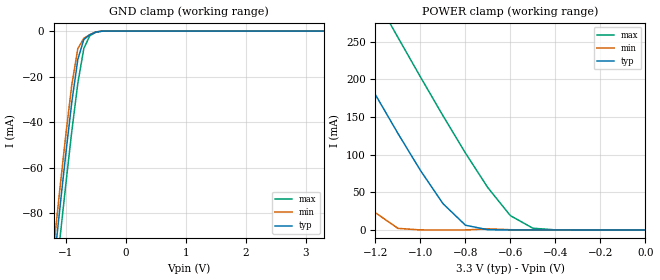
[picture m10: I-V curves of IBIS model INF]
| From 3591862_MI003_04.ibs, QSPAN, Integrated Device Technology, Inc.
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|   Model INF
[Model]   INF
Model_type   Input
Polarity   Non-Inverting
Vinl =   0.8000V
Vinh =   2.0000V
C_comp   5.0000pF   5.0000pF   5.0000pF
[Temperature Range]   27.0000   0.000   70.0000
[Voltage Range]   3.3000V   3.0000V   3.5000V
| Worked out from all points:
|   GND clamp passes 1 mA (typ) near -0.55 V on its own axis
|   POWER clamp passes 1 mA (typ) near -0.71 V on its own axis
[GND_clamp]
| voltage   I(typ)   I(min)   I(max)
-3.3V     -657.8mA   -650mA     -670.4mA
-1.2V     -102.9mA   -94.41mA   -116.5mA
-1.1V     -77.92mA   -69.49mA   -91.49mA
-1V       -53.74mA   -45.47mA   -67.11mA
-900mV    -31.1mA    -23.5mA    -43.83mA
-800mV    -12.43mA   -7.699mA   -22.86mA
-700mV    -3.677mA   -3.173mA   -7.646mA
-600mV    -1.604mA   -1.565mA   -2.006mA
-500mV    -425uA     -358.5uA   -542.4uA
-300mV    -1.113uA   -303.8nA   -5.045uA
3.3V      99.47pA    10.09nA    -13.74uA
[POWER_clamp]
| voltage   I(typ)   I(min)   I(max)
-3.3V     1.331A     1.151A     1.463A
-1.7V     447.3mA    270.6mA    579.2mA
-1.4V     285.1mA    113.5mA    416mA
-1.3V     231.9mA    64.74mA    362.1mA
-1.2V     179.4mA    22.86mA    308.5mA
-1.1V     128mA      2.107mA    255.4mA
-900mV    34.94mA    634.8nA    151.6mA
-800mV    6.306mA    9.188nA    102mA
-700mV    263.5uA    1.485mA    55.91mA
-600mV    6.458uA    324.3uA    18.95mA
-500mV    138.5nA    23.43uA    2.303mA
0V        104.4pA    78.13pA    420.4pA
